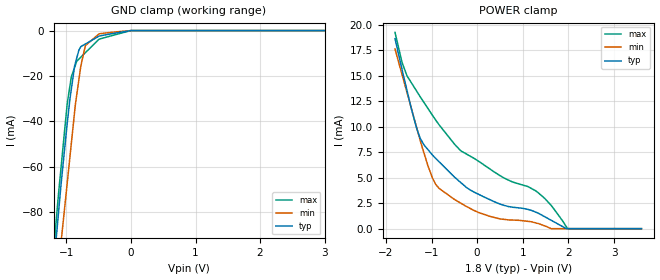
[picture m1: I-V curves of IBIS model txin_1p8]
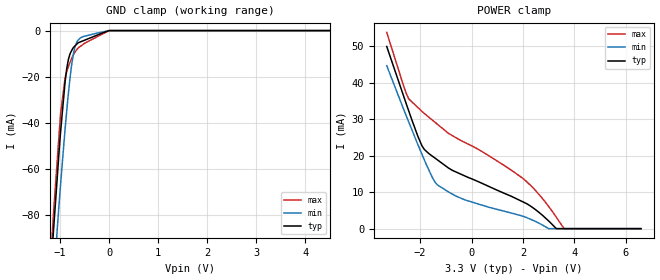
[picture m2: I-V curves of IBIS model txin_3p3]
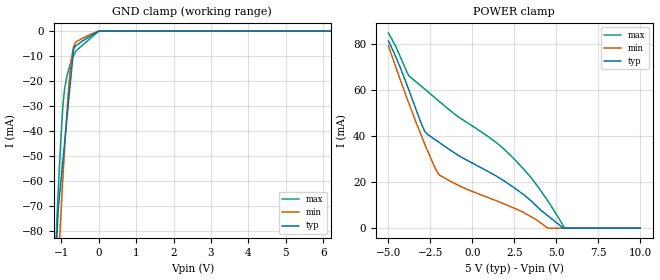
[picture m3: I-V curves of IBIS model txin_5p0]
|Texas Instruments Incorporated
|On-Off Keying Coax Modem Transceivers
| Marketing part#   Digital Voltage Range   Package-type   #pins
| SN65HVD62RGT   1.6V  - 5.5V   QFN   16
| SN65HVD62RGTR   1.6V  - 5.5V   QFN   16
[IBIS Ver]   3.2
[File name]   sn65hvd62.ibs
[File Rev]   1.0
[Date]   5/2/2012
[Source]
| Texas Instruments Incorporated.
| Analog-eLab Design Center, HPA
| 12500 TI Blvd
| Dallas, TX -75243
| e-mail: elab_scm_ibis@list.ti.com
[Notes]   Revision History:
| Rev 1.0: 5/2/2012
| - Initial version of the model
| - Model generated from simulations in TISPICE
| - Model matched to SPICE simulation
| - C_comp although listed in numerical order of value are
|   obtained from varying PVT conditions. For PVT conditions for
|   each specific value refer the buffer description under
|   respective [Model]. IBIS model user is responsible for using
|   appropriate C_comp to simulate for Signal Integrity.
| - Model names with a trailing _1p8 contains the model for
|   1.8V [1.62V and 1.98V].Model names with a trailing _3p3
|   contains the model for 3.3V [3.0V and 3.6V]. Model names with
|   a trailing _5 contains the model for 5.0V [4.5V and 5.5V].
|*  EXCEPTION:   *
|*  - For model txin_*, there will be a leakage current in the power clamp  *
|*   I-V Table because of the resistors in the switches connected to pad.  *
|*  - For model dirset1_*, there will be a leakage current in the power   *
|*   clamp I-V Table because of the series resistor connected to pad.   *
|*  - For model dirset2_*, there will be a leakage current in the power   *
|*   clamp I-V Table because of the series resistor connected to pad.   *
|*  - For model rxo_*, there will be a leakage current in the power clamp   *
|*   I-V Table because of the transistors in the esd connected to pad.   *
[Disclaimer]
| This model is designed as an aid for customers of Texas Instruments.
| TI and its licensors and suppliers make no warranties, either expressed
| or implied, with respect to this  model, including the warranties of
| merchantability or fitness for a particular purpose. The model is
| provided solely on an "as is" basis. The entire risk as to its quality
| and performance is with the customer.
[Copyright]
 (C) Copyright 2012 Texas Instruments Incorporated.All rights reserved.
|   SN65HVD62
[Component]   SN65HVD62
[Manufacturer]   TI
[Package]   |16 QFN   -  RGT package
|   typ   min   max
R_pkg   0.05038   0.02767   0.05471
L_pkg   0.87026nH   0.65097nH   0.92685nH
C_pkg   0.17298pF   0.15490pF   0.19047pF
[Pin]  signal_name   model_name   R_pin   L_pin   C_pin
1   SYNCOUT   SYNC   0.05057   0.85911nH  0.15490pF
2   TXIN   TXIN   0.05337   0.90929nH  0.17853pF
3   VL   POWER   0.05061   0.86318nH  0.17520pF
4   RXOUT   RXO   0.05233   0.89182nH  0.16237pF
5   DIR   DIR   0.05371   0.91260nH  0.15928pF
6   DIRSET2   DIRSET2   0.05089   0.86193nH  0.17714pF
7   DIRSET1   DIRSET1   0.05383   0.91403nH  0.18020pF
8   GND   GND   0.01781   0.53449nH  0.20352pF
9   RES   TERM   0.05065   0.85298nH  0.15578pF
10   BIAS   TERM   0.05471   0.92685nH  0.18135pF
11   RXIN   TERM   0.05220   0.88366nH  0.17772pF
12   TXOUT   TERM   0.02767   0.65097nH  0.19047pF
13   VCC   POWER   0.01732   0.48199nH  0.20330pF
14   XTAL1   TERM   0.05099   0.86507nH  0.17788pF
15   XTAL2   TERM   0.05365   0.91482nH  0.18009pF
16   GND   GND   0.01785   0.53882nH  0.20319pF
|   Model Selectors
[Model Selector] TXIN
txin_1p8  1.8V digital input
txin_3p3  3.3V digital input
txin_5p0  5.0V digital input
[Model Selector] DIRSET2
dirset2_1p8  1.8V digital input
dirset2_3p3  3.3V digital input
dirset2_5p0  5.0V digital input
[Model Selector] DIRSET1
dirset1_1p8  1.8V digital input
dirset1_3p3  3.3V digital input
dirset1_5p0  5.0V digital input
[Model Selector] DIR
dir_1p8  1.8V digital tristate
dir_3p3  3.3V digital tristate
dir_5p0  5.0V digital tristate
[Model Selector] RXO
rxo_1p8  1.8V digital tristate
rxo_3p3  3.3V digital tristate
rxo_5p0  5.0V digital tristate
[Model Selector] SYNC
sync_1p8  1.8V digital Open_drain
sync_3p3  3.3V digital Open_drain
sync_5p0  5.0V digital Open_drain
[Model Selector] TERM
term_1-8V  1.8V nominal termination
term_3-3V  3.3V nominal termination
term_5-0V  5.0V nominal termination
[Model] term_1-8V
Model_type Terminator
C_comp   1.0e-20F  1.0e-20F  1.0e-20F
|   typ   min   max
[Voltage Range]   1.8V   1.62V   1.98V
[POWER Clamp Reference]   1.8V   1.62V   1.98V
[GND Clamp Reference]   0V   0V   0V
|Ambient Temperature   25   85   -40
|Junction Temperature
[Temperature Range]   27   125   -40
[Model] term_3-3V
Model_type Terminator
C_comp   1.0e-20F  1.0e-20F  1.0e-20F
|   typ   min   max
[Voltage Range]   3.3V   3.0V   3.6V
[POWER Clamp Reference]   3.3V   3.0V   3.6V
[GND Clamp Reference]   0V   0V   0V
|Ambient Temperature   25   85   -40
|Junction Temperature
[Temperature Range]   27   125   -40
[Model] term_5-0V
Model_type Terminator
C_comp   1.0e-20F  1.0e-20F  1.0e-20F
|   typ   min   max
[Voltage Range]   5.0V   4.5V   5.5V
[POWER Clamp Reference]   5.0V   4.5V   5.5V
[GND Clamp Reference]   0V   0V   0V
|Ambient Temperature   25   85   -40
|Junction Temperature
[Temperature Range]   27   125   -40
| Models and submodels in the file (21): txin_1p8 (Input), txin_3p3 (Input), txin_5p0 (Input), dirset2_1p8 (Input), dirset2_3p3 (Input), dirset2_5p0 (Input), dirset1_1p8 (Input), dirset1_3p3 (Input), dirset1_5p0 (Input), dir_1p8 (3-state), dir_3p3 (3-state), dir_5p0 (3-state), rxo_1p8 (3-state), rxo_3p3 (3-state), rxo_5p0 (3-state), sync_1p8 (Open_drain), sync_3p3 (Open_drain), sync_5p0 (Open_drain), term_1-8V (Terminator), term_3-3V (Terminator), term_5-0V (Terminator)
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|   txin_1p8 Model
[Model]   txin_1p8
Model_type   Input
Vinl = 0.54
Vinh = 1.26
|   typ   min   max
 C_comp   7.669e-13   7.486e-13   7.832e-13
| Where nom  PVT is Nominal Process, 1.8V, 27C
|   Fast PVT is Strong Process,  1.98V, -40C
|   Slow PVT is Weak Process,   1.62V, 125C
[Voltage Range]   1.8   1.62   1.98
|Ambient Temperature   25   85   -40
|Junction Temperature
[Temperature Range]   27   125   -40
[Power Clamp Reference]   1.8   1.62   1.98
[GND Clamp Reference]   0   0   0
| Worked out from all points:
|   GND clamp passes 1 mA (typ) near -0.22 V on its own axis
[GND Clamp]
|   Voltage   I(typ)   I(min)   I(max)
-1.8V     -315.1mA   -322.3mA   -323.5mA
-1.265V   -125.8mA   -149.1mA   -120.6mA
-1.158V   -91.69mA   -115mA     -83.79mA
-1.087V   -69.05mA   -94.52mA   -61.55mA
-986mV    -40.43mA   -66.77mA   -31.89mA
-924.7mV  -25.93mA   -49.93mA   -20.44mA
-873mV    -15.58mA   -35.76mA   -16.22mA
-777.6mV  -7.096mA   -15.7mA    -11.75mA
-706.3mV  -5.921mA   -6.633mA   -9.751mA
-494.1mV  -2.434mA   -1.434mA   -3.811mA
-29.03fV  -180nA     -178.5nA   -208.1nA
3.6V      0A         0A         0A
[POWER Clamp]
|   Voltage   I(typ)   I(min)   I(max)
-1.8V     18.66mA    17.63mA    19.26mA
-1.645V   15.61mA    15.12mA    16.31mA
-1.538V   13.59mA    13.38mA    15.01mA
-1.251V   8.899mA    8.708mA    12.97mA
-983.3mV  7.255mA    5.017mA    11.15mA
-837.5mV  6.584mA    3.967mA    10.22mA
-360.4mV  4.531mA    2.505mA    7.652mA
-72mV     3.601mA    1.793mA    6.913mA
601.9mV   2.273mA    904.7uA    4.942mA
1.329V    1.543mA    511.8uA    3.563mA
1.982V    0A         0A         0A
3.6V      0A         0A         0A
|   txin_3p3 Model
[Model]   txin_3p3
Model_type   Input
Vinl = 0.99
Vinh = 2.3
|   typ   min   max
 C_comp   6.859e-13   6.748e-13   6.882e-13
| Where nom  PVT is Nominal Process, 3.3V, 27C
|   Fast PVT is Strong Process,  3.6V, -40C
|   Slow PVT is Weak Process,   3V, 125C
[Voltage Range]   3.3   3   3.6
|Ambient Temperature   25   85   -40
|Junction Temperature
[Temperature Range]   27   125   -40
[Power Clamp Reference]   3.3   3   3.6
[GND Clamp Reference]   0   0   0
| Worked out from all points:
|   GND clamp passes 1 mA (typ) near -0.13 V on its own axis
[GND Clamp]
|   Voltage   I(typ)   I(min)   I(max)
-3.3V     -890.5mA   -851.4mA   -944.2mA
-1.195V   -104.8mA   -126.5mA   -99.66mA
-1.127V   -84.35mA   -106.4mA   -76.72mA
-1.032V   -55.76mA   -78.26mA   -48.4mA
-990mV    -43.84mA   -66.55mA   -35.85mA
-896.4mV  -21.86mA   -42.15mA   -20.2mA
-864.6mV  -16.49mA   -34.7mA    -17.86mA
-801mV    -10.35mA   -21.15mA   -13.96mA
-720mV    -7.136mA   -9.15mA    -10.15mA
-534mV    -4.449mA   -2.629mA   -6.003mA
-33.83fV  -329.9nA   -328.9nA   -378.4nA
6.6V      0A         0A         0A
[POWER Clamp]
|   Voltage   I(typ)   I(min)   I(max)
-3.3V     49.95mA    44.69mA    53.83mA
-2.668V   36.87mA    33.2mA     39.67mA
-2.444V   32.3mA     29.28mA    35.61mA
-1.927V   22.69mA    20.38mA    32.15mA
-1.539V   19.96mA    14.25mA    29.86mA
-1.329V   18.87mA    12.01mA    28.64mA
-285mV    14.54mA    7.976mA    23.73mA
2.038V    7.222mA    3.317mA    13.55mA
3.003V    2.118mA    0A         6.099mA
3.303V    0A         0A         3.113mA
3.604V    0A         0A         0A
6.6V      0A         0A         0A
|   txin_5p0 Model
[Model]   txin_5p0
Model_type   Input
Vinl = 1.5
Vinh = 3.5
|   typ   min   max
 C_comp   6.210e-13   6.152e-13   6.249e-13
| Where nom  PVT is Nominal Process, 5V, 27C
|   Fast PVT is Strong Process,  5.5V, -40C
|   Slow PVT is Weak Process,   4.5V, 125C
[Voltage Range]   5   4.5   5.5
|Ambient Temperature   25   85   -40
|Junction Temperature
[Temperature Range]   27   125   -40
[Power Clamp Reference]   5   4.5   5.5
[GND Clamp Reference]   0   0   0
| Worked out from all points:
|   GND clamp passes 1 mA (typ) near -0.11 V on its own axis
[GND Clamp]
|   Voltage   I(typ)   I(min)   I(max)
-5V       -1.56A     -1.481A    -1.656A
-1.14V    -89.35mA   -111.1mA   -83.49mA
-1.111V   -80.5mA    -102.2mA   -73.31mA
-1.08V    -71.04mA   -92.73mA   -63.7mA
-1.023V   -62.13mA   -76.83mA   -46.22mA
-962.5mV  -52.68mA   -60.09mA   -31.14mA
-913mV    -44.94mA   -47.6mA    -23.31mA
-801mV    -27.44mA   -22.08mA   -15.38mA
-684mV    -9.163mA   -7.028mA   -10.08mA
-605mV    -5.837mA   -4.255mA   -7.947mA
-84.44fV  -499.8nA   -492.3nA   -578.1nA
10V       0A         0A         0A
[POWER Clamp]
|   Voltage   I(typ)   I(min)   I(max)
-5V       81.48mA    79.3mA     84.91mA
-4.543V   74.23mA    69.77mA    78.76mA
-3.773V   59.94mA    54.16mA    66.2mA
-2.84V    42.15mA    36.68mA    60.51mA
-2.245V   38.65mA    26.6mA     56.83mA
-1.958V   37.2mA     23.09mA    55.05mA
1.254V    23.39mA    12.44mA    38.2mA
2.376V    18.15mA    9.05mA     30.97mA
3.547V    11.51mA    4.801mA    21.53mA
4.505V    5.39mA     0A         11.83mA
5.505V    0A         0A         0A
10V       0A         0A         0A
